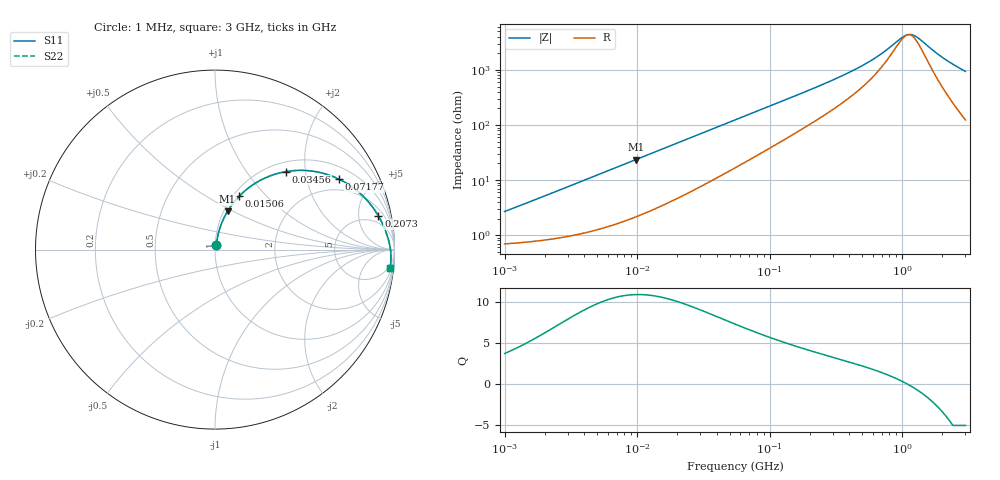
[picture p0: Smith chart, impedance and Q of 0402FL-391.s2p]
# MHz S MA R 50
!Freq  MagS11  AngS11  MagS21  AngS21  MagS12  AngS12  MagS22  AngS22
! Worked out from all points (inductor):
!   801 points, 1 MHz to 3 GHz, reference 50 ohm
!   read as one part in series: L = 409 nH near 1.041 MHz
!   highest Q = 10.9 at 9.794 MHz (marker M1), where L = 381 nH
!   self-resonance near 1.106 GHz
!   S11 on the Smith chart (normalised r, x): 1 MHz: 1.01, +0.05; 15.06 MHz: 1.07, +0.71; 34.56 MHz: 1.18, +1.57; 71.77 MHz: 1.48, +3.15; 207.3 MHz: 3.15, +8.71; 3 GHz: 3, -19
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1  0.02664 73.6  0.9928 -1.5  0.9928 -1.5  0.02664 73.6
3.823119  0.09387 78.2  0.9852 -5.4  0.9852 -5.4  0.09387 78.2
9.794439  0.2246 71.8  0.9542 -12.9  0.9542 -12.9  0.2246 71.8
14.47069  0.3152 66.4  0.9201 -18.3  0.9201 -18.3  0.3152 66.4
15.06173  0.3258 65.7  0.9154 -18.9  0.9154 -18.9  0.3258 65.7
22.47661  0.4453 57.9  0.8514 -26.3  0.8514 -26.3  0.4453 57.9
34.56417  0.5882 47.7  0.744 -35.8  0.744 -35.8  0.5882 47.7
54.77226  0.7292 36.0  0.5929 -46.3  0.5929 -46.3  0.7292 36.0
71.76513  0.7951 29.5  0.4987 -51.8  0.4987 -51.8  0.7951 29.5
118.3678  0.8794 19.5  0.3403 -59.8  0.3403 -59.8  0.8794 19.5
207.3156  0.9299 11.6  0.2072 -64.5  0.2072 -64.5  0.9299 11.6
209.4008  0.9305 11.5  0.2053 -64.6  0.2053 -64.6  0.9305 11.5
328.5236  0.952 7.2  0.1311 -65.0  0.1311 -65.0  0.952 7.2
471.0174  0.963 4.6  0.08685 -62.5  0.08685 -62.5  0.963 4.6
623.3561  0.9692 2.9  0.05904 -57.1  0.05904 -57.1  0.9692 2.9
792.5923  0.9733 1.7  0.03911 -46.1  0.03911 -46.1  0.9733 1.7
1028.15  0.9768 0.4  0.02397 -14.8  0.02397 -14.8  0.9768 0.4
1113.852  0.9778 -0.0  0.02225 1.6  0.02225 1.6  0.9778 -0.0
1194.682  0.9785 -0.4  0.02251 16.9  0.02251 16.9  0.9785 -0.4
1333.714  0.9795 -0.9  0.02613 37.9  0.02613 37.9  0.9795 -0.9
2071.593  0.9819 -3.4  0.06098 71.0  0.06098 71.0  0.9819 -3.4
3000  0.981 -5.9  0.104 76.5  0.104 76.5  0.981 -5.9
